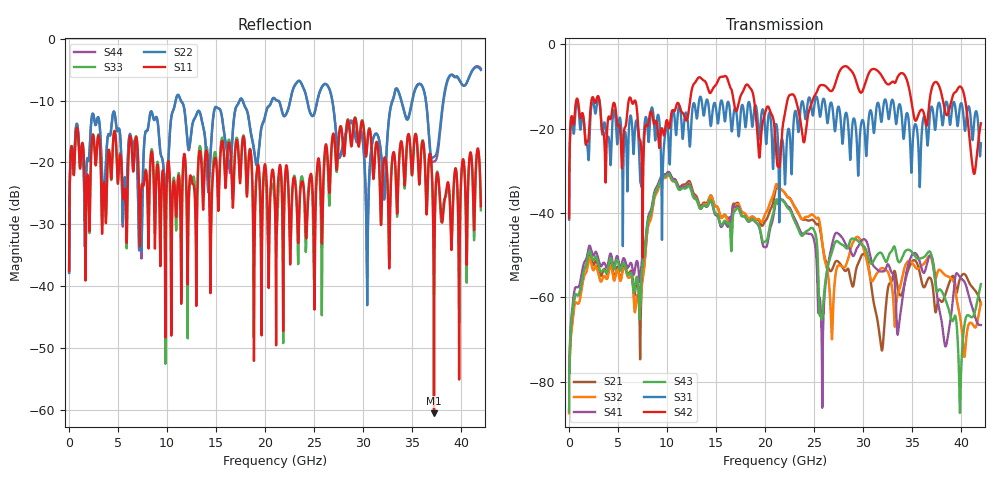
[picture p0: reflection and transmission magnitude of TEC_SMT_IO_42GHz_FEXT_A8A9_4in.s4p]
!! CHANNEL DESCRIPTION: Next Generation 28Gbps High Density SMT I/O Connector
!!  with 4" 5-6-5 Megatron 6 Stripline trace on host side and 1.25" 7-5-7 Megtron 6 Microstrip trace on plug side at 14GHz
!! HOST PCB DESCRIPTION: PCB thickness 2.86 mm, Nelco 4000-13SI (Dk 3.32, Df 0.010)
!!  23 Layer Board, 12 GND planes, 2 Layer route-out on Layers 10,12, 8 mil stub on vias
!!  Pairs on following layers
!!  Layer 10 - A8A9
!! CONNECTOR DESCRIPTION:  Next Generation 28Gbps High Density SMT I/O Connector
!! PLUG-IN CARD DESCRIPTION:  PCB thickness 1mm thick, Nelco 4000-13SI (Dk 3.32, Df 0.010)
!!  6 Layer Board, 4 GND planes, 0.35 x 1.4mm mating pads
!!  Micro-strip diff traces referenced to GND plane 3mils down, 2nd GND plane 15mils from top of board
!!  PCB GND planes are symmetric
!! MODEL DESCRIPTION: TE Connectivity S-parameter model produced from Macro-model
!! MODEL DATE: 9/25/2014 CR1a_GC1i, VR6&12_4
!! MODEL STATUS: Developmental
!! MODEL GEOMETRY: 2 Rows - Rows A, B. 3 pairs in each row, 6 total pairs
!! MODEL FREQUENCY RANGE: DC to 42 GHz in 10 MHz frequency steps
!! MODEL EDGE RATE LIMITATION: 11.90 ps (Using conservative 0.5/Fmax rule of thumb)
!! TIME-DOMAIN TRANSFORM CAUTIONS:
!! 1.) Do not simulate transient edge rates faster than the number listed above.  Edge
!!  rates faster than this number contain significant spectral content at frequencies
!!  above the model's highest frequency.
!! 2.) Even when simulating edge rates that are slower than the number listed above, be
!!  aware that the best time resolution possible with a direct iFFT is (1 / 2Fmax).
!!  As a result, time resolution is typically not adequate for most time-domain
!!  simulations unless tricks such as frequency-domain zero-padding and windowing are
!!  used to minimize leakage and aliasing.
!! 3.) Because the model has a uniform frequency step, a direct iFFT will result in an
!!  impulse that that has a time length given by either (1 / Fstep) or (1 / 2Fstep),
!!  depending on the transform being used.  Care has been taken in selecting the
!!  frequency step to ensure a settled impulse response for the model.  Therefore,
!!  convolution with the model's impulse response should present no issues.  However,
!!  if directly concatenating s-parameter models in the frequency domain a user must
!!  either interpolate necessary interim frequencies or complete impulse response
!!  zero-padding.  Impulse response zero-padding is more difficult, but more accurate.
!! PORT DEFINITIONS:
!! Port  1  ----->  Host, Bot Row  A8  B5  Module, Top Row  <-----  Port  2
!! Port  3  ----->  Host, Bot Row  A9  B6  Module, Top Row  <-----  Port  4
# Hz S MA R 50
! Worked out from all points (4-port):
!   4200 points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, 10 MHz to 42 GHz, reference 50 ohm
!   strongest paths, dB at 10 MHz, 10.51 GHz, 21.01 GHz, 31.51 GHz, 42 GHz:
!     S42: -41.1, -15.7, -21.2, -6.3, -18.7
!     S31: -41.5, -16.6, -20.0, -13.8, -23.4
!     S43: -87.1, -32.2, -37.8, -49.7, -56.8
!     S41: -86.8, -31.7, -38.3, -53.6, -66.5
!     S32: -87.5, -32.3, -34.0, -53.9, -61.3
!     S21: -87.2, -31.7, -35.1, -66.2, -61.6
!   lowest |S11| = -60.6 dB at 37.22 GHz (marker M1), VSWR 1.00, Z = 49.9 - j0.0202 ohm
!   |S11| at or under -10 dB: start of sweep to end of sweep
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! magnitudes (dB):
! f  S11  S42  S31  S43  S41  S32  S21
! 10 MHz  -37.5  -41.1  -41.5  -87.1  -86.8  -87.5  -87.2
! 10.1 GHz  -19.8  -18.9  -21.1  -30.7  -30.2  -31.0  -30.4
! 21.87 GHz  -36.4  -18.2  -25.0  -37.2  -37.0  -34.8  -34.8
! 25.81 GHz  -32.7  -9.6  -14.0  -64.9  -81.7  -46.6  -47.0
! 37.22 GHz  -60.6  -9.1  -18.2  -53.7  -52.9  -54.0  -60.3
! 39.88 GHz  -28.2  -10.0  -14.6  -86.8  -55.3  -64.7  -55.5
! 42 GHz  -27.1  -18.7  -23.4  -56.8  -66.5  -61.3  -61.6
